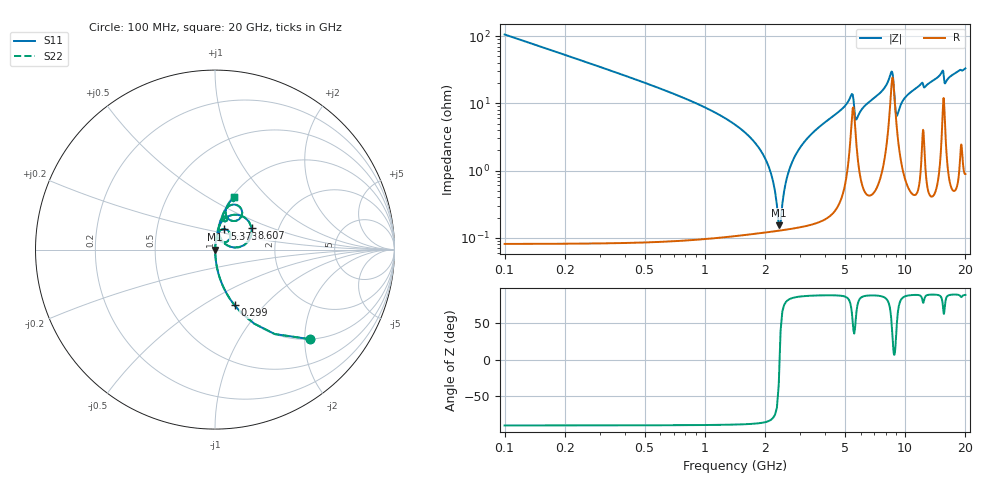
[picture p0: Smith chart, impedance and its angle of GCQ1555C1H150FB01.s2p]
!Murata Part Number: GCQ1555C1H150FB01
!These Parameters are Measured in Series Mode Connection
!Data Generated on Jan 08, 2026
!  o--ll--o
!Port1  Port2
!  o------o
!Operation Temp=25[degC], DC Bias Voltage=0[V]
!Freq. Start=100[MHz] Stop=20[GHz] 401[Steps]
# Hz S RI R 50
!Freq.(Hz) S11(Real) S11(Imag) S21(Real) S21(Imag) S12(Real) S12(Imag) S22(Real) S22(Imag)
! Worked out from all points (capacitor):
!   401 points, 100 MHz to 20 GHz, reference 50 ohm
!   read as one part in series: C = 15 pF near 199.5 MHz
!   lowest |Z| = 154 mohm at 2.339 GHz (marker M1)
!   series resonance near 2.361 GHz, so ESL is about 300 pH
!   S11 on the Smith chart (normalised r, x): 100 MHz: 1.00, -2.12; 299 MHz: 1.00, -0.70; 5.373 GHz: 1.08, +0.25; 8.607 GHz: 1.45, +0.38; 20 GHz: 1.02, +0.66
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1e8  0.5287 -0.4988  0.4713 0.4988  0.4713 0.4988  0.5287 -0.4988
2.99e8  0.1093 -0.3108  0.8907 0.3108  0.8907 0.3108  0.1093 -0.3108
7.965e8  0.0146 -0.1163  0.9854 0.1163  0.9854 0.1163  0.0146 -0.1163
1.891e9  0.00158 -0.0202  0.9984 0.0202  0.9984 0.0202  0.00158 -0.0202
2.09e9  0.00134 -0.0111  0.9987 0.0111  0.9987 0.0111  0.00134 -0.0111
2.33875e9  0.00127 -0.000861  0.9987 0.000861  0.9987 0.000861  0.00127 -0.000861
2.43825e9  0.0013 0.00292  0.9987 -0.00292  0.9987 -0.00292  0.0013 0.00292
2.5875e9  0.0014 0.00835  0.9986 -0.00835  0.9986 -0.00835  0.0014 0.00835
2.7865e9  0.00161 0.0152  0.9984 -0.0152  0.9984 -0.0152  0.00161 0.0152
3.43325e9  0.00284 0.0356  0.9972 -0.0356  0.9972 -0.0356  0.00284 0.0356
5.3735e9  0.0529 0.1137  0.9471 -0.1137  0.9471 -0.1137  0.0529 0.1137
5.72175e9  0.0252 0.0504  0.9748 -0.0504  0.9748 -0.0504  0.0252 0.0504
6.7665e9  0.0162 0.1084  0.9838 -0.1084  0.9838 -0.1084  0.0162 0.1084
8.06e9  0.0538 0.1725  0.9462 -0.1725  0.9462 -0.1725  0.0538 0.1725
8.60725e9  0.2036 0.1231  0.7964 -0.1231  0.7964 -0.1231  0.2036 0.1231
9.055e9  0.0484 0.0391  0.9516 -0.0391  0.9516 -0.0391  0.0484 0.0391
1.005e10  0.0218 0.1204  0.9782 -0.1204  0.9782 -0.1204  0.0218 0.1204
1.338325e10  0.0444 0.1962  0.9556 -0.1962  0.9556 -0.1962  0.0444 0.1962
1.53235e10  0.117 0.2495  0.883 -0.2495  0.883 -0.2495  0.117 0.2495
1.5821e10  0.0778 0.1685  0.9222 -0.1685  0.9222 -0.1685  0.0778 0.1685
1.67165e10  0.0633 0.2303  0.9367 -0.2303  0.9367 -0.2303  0.0633 0.2303
2e10  0.1052 0.2937  0.8948 -0.2937  0.8948 -0.2937  0.1052 0.2937
